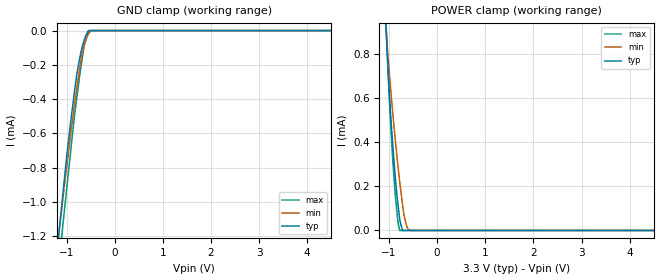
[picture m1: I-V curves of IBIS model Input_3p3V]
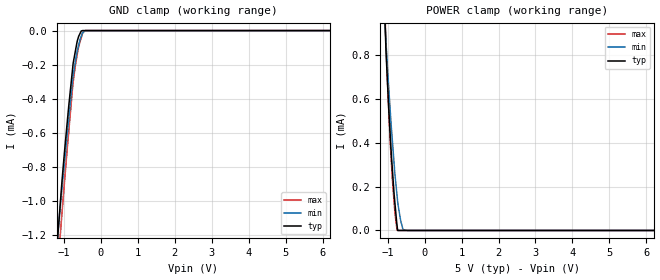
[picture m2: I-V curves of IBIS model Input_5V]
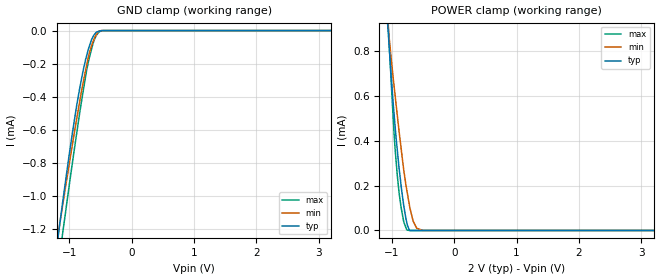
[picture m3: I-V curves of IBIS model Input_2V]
| Texas Instruments Incorporated
| 16-Bit, Quad Channel, Ultra-Low Glitch, Voltage Output DAC with 2.5V,
| 2ppm/C Internal Reference
| Marketing part#   Voltage Range   Package-type   #pins
| DAC8564IAPW   1.8 to 5.5V   TSSOP   16
| DAC8564IAPWG4   1.8 to 5.5V   TSSOP   16
| DAC8564IAPWR   1.8 to 5.5V   TSSOP   16
| DAC8564IAPWRG4   1.8 to 5.5V   TSSOP   16
| DAC8564IBPW   1.8 to 5.5V   TSSOP   16
| DAC8564IBPWG4   1.8 to 5.5V   TSSOP   16
| DAC8564IBPWR   1.8 to 5.5V   TSSOP   16
| DAC8564IBPWRG4   1.8 to 5.5V   TSSOP   16
| DAC8564ICPW   1.8 to 5.5V   TSSOP   16
| DAC8564ICPWG4   1.8 to 5.5V   TSSOP   16
| DAC8564ICPWR   1.8 to 5.5V   TSSOP   16
| DAC8564ICPWRG4   1.8 to 5.5V   TSSOP   16
| DAC8564IDPW   1.8 to 5.5V   TSSOP   16
| DAC8564IDPWG4   1.8 to 5.5V   TSSOP   16
| DAC8564IDPWR   1.8 to 5.5V   TSSOP   16
| DAC8564IDPWRG4   1.8 to 5.5V   TSSOP   16
[IBIS Ver]   3.2
[File name]   dac8564.ibs
|SIMDE Ver   V2.0 - 201002 - RHL4 - Build 372
[Date]   29 July 2010
[File Rev]   1.2
[Source]
| Texas Instruments Incorporated.
| Analog eLab Design Center, HPA
| 12500 TI Blvd
| Dallas, TX -75243
| e-Mail: elab_scm_ibis@list.ti.com
| Model generated from simulations in TISPICE
[Notes]Revision_History:
|   Rev 1.0: 06/08/2010
|   - Initial version of the model
|   - Model names with a trailing _2p25V stands for the Model
|   with typical voltage 2.25V -[1.8V,2.25V,2.7V].Model names
|   with a trailing _4p1V stands for the Model with typical
|   voltage 4.1V-[2.7V,4.1V,5.5V]
|   Rev 1.1: 07/08/2010
|   - Model generated from simulations in TISPICE
|   - Model matched to SPICE simulation
|   - Updated the ibis file with data sheet title and package
|   details
|   - While calculating R_pkg, L_pkg and C_pkg ignored values
|   corresponding to power and ground pins
|   - Added package details beside [Package]
|   - Re-genearted the Models with std typical values of 3.3V
|   and 5V . The 2 Models are
|   1) Input_3p3V - corresponds to 3V  , 3.3V,3.6V
|   2) Input_5V   - corresponds to 4.5V, 5V  ,5.5V
|   - C_comp although listed in numerical order of value are
|   obtained from varying PVT conditions. For PVT conditions
|   for each specific value refer the buffer description under
|   respective [Model]. IBIS model user is responsible for using
|   appropriate C_comp to simulate for Signal Integrity
|   Rev 1.2: 07/08/2010
|   - Corrected Vinl and Vinh for all models
|   - Removed all points beyond rail voltages
|   - Used 1.0E-20F for C_comp of TERM
|   - Corrected the typical value calculation for package RLC
[Disclaimer]
| This model is designed as an aid for customers of Texas Instruments.
| TI and its licensors and suppliers make no warranties, either expressed
| or implied, with respect to this  model, including the warranties of
| merchantability or fitness for a particular purpose. The model is
| provided solely on an "as is" basis. The entire risk as to its quality
| and performance is with the customer.
[Copyright]
| (C) Copyright 2010 Texas Instruments Incorporated. All rights reserved.
|   DAC8564
[Component]   DAC8564
[Manufacturer]  TI
[Package] | 16 TSSOP - PW package
|   typ   min   max
R_pkg   0.05811   0.02779   0.08182
L_pkg   2.21350E-09   1.70135E-09   2.86250E-09
C_pkg   0.47245E-12   0.44143E-12   0.51313E-12
|-------------------------PINS------------------------------------------------
[Pin]  signal_name   model_name   R_pin   L_pin   C_pin
1   VOUT_A   NC   0.04433   2.55695E-09   0.51313E-12
2   VOUT_B   NC   0.04120   1.94352E-09   0.46611E-12
3   VREF_H/VREF_OUT term   0.02779   1.70135E-09   0.50494E-12
4   AVDD   POWER   0.02688   1.68698E-09   0.49746E-12
5   VREF_L   term   0.03604   1.75816E-09   0.47239E-12
6   GND   GND   0.02752   1.74852E-09   0.49261E-12
7   VOUT_C   NC   0.04259   1.98332E-09   0.46901E-12
8   VOUT_D   NC   0.04432   2.56006E-09   0.51267E-12
9   _SYNC   Input   0.07777   2.80109E-09   0.49072E-12
10   SCLK   Input   0.07962   2.26331E-09   0.44148E-12
11   DIN   Input   0.06860   2.06333E-09   0.44715E-12
12   IOVDD   POWER   0.03580   1.75989E-09   0.46496E-12
13   A0   Input   0.06309   1.96557E-09   0.44143E-12
14   A1   Input   0.06860   2.05920E-09   0.44679E-12
15   _ENABLE   Input   0.07962   2.25708E-09   0.44154E-12
16   LDAC   Input   0.08182   2.86250E-09   0.49444E-12
|   Model Selectors
[Model selector] Input
 Input_3p3V   3.3V nominal input
 Input_5V   5V   nominal input
 Input_2V   2V nominal input
|NOTES   Model Selector is used to select between the Input Models which
|   have 3 Voltage ranges namely
|   1) Input_2V   -  1.8,2,2.2V
|   2) Input_3p3V -  3,3.3,3.6V
|   3) Input_5V   -  4.5,5,5.5V
[Model selector] term
 term_3p3V  3.3V nominal termination
 term_5V   5V   nominal termination
 term_2V   2V   nominal termination
|   Termination - term_3p3V
[Model] term_3p3V
Model_type Terminator
C_comp  1.0E-20F 1.0E-20F 1.0E-20F
| variable   typ   min   max
[Voltage Range]   3.30000v  3.00000V  3.60000V
[POWER Clamp Reference]  3.30000v  3.00000V  3.60000V
[GND Clamp Reference]   0.00000V  0.00000V  0.00000V
[Temperature Range]   25   105   -40
|   Termination - term_5V
[Model] term_5V
Model_type Terminator
C_comp  1.0E-20F 1.0E-20F 1.0E-20F
| variable   typ   min   max
[Voltage Range]   5.00000V  4.50000V  5.50000V
[POWER Clamp Reference]  5.00000V  4.50000V  5.50000V
[GND Clamp Reference]   0.00000V  0.00000V  0.00000V
[Temperature Range]   25   105   -40
|   Termination - term_2V
[Model] term_2V
Model_type Terminator
C_comp  1.0E-20F 1.0E-20F 1.0E-20F
| variable   typ   min   max
[Voltage Range]   2.00000V  1.80000V  2.20000V
[POWER Clamp Reference]  2.00000V  1.80000V  2.20000V
[GND Clamp Reference]   0.00000V  0.00000V  0.00000V
[Temperature Range]   25   105   -40
| Models and submodels in the file (6): Input_3p3V (Input), Input_5V (Input), Input_2V (Input), term_3p3V (Terminator), term_5V (Terminator), term_2V (Terminator)
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|NOTES   Three separate Terminators are modelled for the 3 range of
|   voltages
|   1) term_3p3V -  3,3.3,3.6V
|   2) term_5V   -  4.5,5,5.5V
|   3) term_2p5V -  1.8,2,2.2V
|   Model   - Input_3p3V
[Model]   Input_3p3V
Model_type   Input
Vinl = 0.99
Vinh = 2.31
|   typ   min   max
|   (nom PVT)   (Fast PVT)   (slow PVT)
C_comp   4.648e-13   4.575e-13   5.349e-13
| Where   nom  PVT is  Nominal Process, 3.3V, 25C
|   Fast PVT is Strong Process, 3.6V, -40C
|   Slow PVT is Weak Process, 3.0V, 105C
[model spec]
Vinl   0.99   0.9   1.08
Vinh   2.31   2.1   2.52
[Voltage Range]   3.3   3   3.6
|Ambient Temperature   25   105   -40
|Junction Temperature
[Temperature Range]   25   105   -40
[Power Clamp Reference]   3.3   3   3.6
[GND Clamp Reference]   0   0   0
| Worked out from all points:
|   GND clamp passes 1 mA (typ) near -1.09 V on its own axis
|   POWER clamp passes 1 mA (typ) near -1.08 V on its own axis
[GND Clamp]
|   Voltage   I(typ)   I(min)   I(max)
-3.3V     -7.771mA   -6.599mA   -9.241mA
-1.178V   -1.239mA   -1.228mA   -1.424mA
-1.079V   -961uA     -989.1uA   -1.143mA
-986.7mV  -708.8uA   -773.2uA   -897.2uA
-910.8mV  -524.5uA   -596.9uA   -694.5uA
-834mV    -353.1uA   -431.1uA   -497.2uA
-785.4mV  -253uA     -332.6uA   -390.9uA
-693mV    -117.5uA   -156.6uA   -198.1uA
-636mV    -59.22uA   -87.82uA   -94.01uA
-549.6mV  -492.7nA   -23.01uA   -15.28uA
-471.9mV  0A         0A         0A
6.6V      0A         0A         0A
[POWER Clamp]
|   Voltage   I(typ)   I(min)   I(max)
-3.3V     13.63mA    11.23mA    16.39mA
-1.076V   970.6uA    953.2uA    1.029mA
-1.036V   801.6uA    830uA      786.9uA
-983.4mV  583.8uA    687.3uA    551.2uA
-916.8mV  371.6uA    519.3uA    300uA
-866.4mV  233.2uA    401.4uA    151.6uA
-816mV    122.3uA    293.9uA    42.15uA
-778.8mV  53.33uA    221.7uA    0A
-719.4mV  0A         118.1uA    0A
-672mV    0A         53.15uA    0A
-546mV    0A         0A         0A
6.6V      0A         0A         0A
|   Model   - Input_5V
[Model]   Input_5V
Model_type   Input
Vinl = 1.5
Vinh = 3.5
|   typ   min   max
|   (nom PVT)   (Fast PVT)   (slow PVT)
C_comp   4.340e-13   3.990e-13   5.345e-13
| Where   nom  PVT is  Nominal Process, 5V, 25C
|   Fast PVT is Strong Process, 5.5V, -40C
|   Slow PVT is Weak Process, 4.5V, 105C
[model spec]
Vinl   1.5   1.35   1.65
Vinh   3.5   3.15   3.85
[Voltage Range]   5   4.5   5.5
|Ambient Temperature   25   105   -40
|Junction Temperature
[Temperature Range]   25   105   -40
[Power Clamp Reference]   5   4.5   5.5
[GND Clamp Reference]   0   0   0
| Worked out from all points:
|   GND clamp passes 1 mA (typ) near -1.09 V on its own axis
|   POWER clamp passes 1 mA (typ) near -1.08 V on its own axis
[GND Clamp]
|   Voltage   I(typ)   I(min)   I(max)
-5V       -13.07mA   -10.95mA   -15.71mA
-1.155V   -1.177mA   -1.174mA   -1.362mA
-1.079V   -959.1uA   -987.9uA   -1.144mA
-990mV    -726.1uA   -787.4uA   -903.6uA
-870mV    -444.5uA   -519.3uA   -594.1uA
-750mV    -191.7uA   -263.6uA   -301.6uA
-640mV    -62.84uA   -120.2uA   -140.6uA
-600mV    -33uA      -83.78uA   -92.78uA
-530mV    -2.078uA   -32.4uA    -41.23uA
-490mV    0A         -10.72uA   -13.32uA
-423.5mV  0A         0A         0A
10V       0A         0A         0A
[POWER Clamp]
|   Voltage   I(typ)   I(min)   I(max)
-5V       23.6mA     19.51mA    28.37mA
-1.094V   1.06mA     1.017mA    1.141mA
-1.056V   876.4uA    897.1uA    904.7uA
-990.5mV  625.8uA    702.1uA    620uA
-930mV    430uA      543.8uA    402.5uA
-869.5mV  270.8uA    401.9uA    226.7uA
-798mV    114.6uA    247.1uA    72.56uA
-745mV    20.34uA    157.4uA    1.195uA
-729.5mV  581.7nA    131.2uA    0A
-594.5mV  0A         10.2uA     0A
-451.5mV  0A         0A         0A
10V       0A         0A         0A
|   Model   - Input_2V
[Model]   Input_2V
Model_type   Input
Vinl = 0.2
Vinh = 1.9
|   typ   min   max
|   (nom PVT)   (Fast PVT)   (slow PVT)
C_comp   4.997e-13   4.480e-13   5.391e-13
| Where   nom  PVT is  Nominal Process, 2V, 25C
|   Fast PVT is Strong Process, 2.2V, -40C
|   Slow PVT is Weak Process, 1.8V, 105C
[model spec]
Vinl   0.2   0.18   0.22
Vinh   1.9   1.71   2.09
[Voltage Range]   2   1.8   2.2
|Ambient Temperature   25   105   -40
|Junction Temperature
[Temperature Range]   25   105   -40
[Power Clamp Reference]   2   1.8   2.2
[GND Clamp Reference]   0   0   0
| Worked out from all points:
|   GND clamp passes 1 mA (typ) near -1.09 V on its own axis
|   POWER clamp passes 1 mA (typ) near -1.09 V on its own axis
[GND Clamp]
|   Voltage   I(typ)   I(min)   I(max)
-2V       -3.727mA   -3.282mA   -4.306mA
-1.168V   -1.212mA   -1.204mA   -1.397mA
-1.108V   -1.039mA   -1.059mA   -1.228mA
-944mV    -601.3uA   -672.3uA   -780.8uA
-878mV    -443uA     -523.6uA   -608.9uA
-782mV    -247.4uA   -320.5uA   -374.3uA
-721.8mV  -150.5uA   -208.1uA   -237.8uA
-684.4mV  -99.5uA    -143.7uA   -171uA
-620.6mV  -36.88uA   -66.41uA   -78.82uA
-558mV    -7.517uA   -17.35uA   -24.33uA
-454mV    0A         0A         0A
4V        0A         0A         0A
[POWER Clamp]
|   Voltage   I(typ)   I(min)   I(max)
-2V       6.043mA    4.961mA    7.255mA
-1.066V   914uA      922.6uA    963.1uA
-1.041V   809.3uA    851uA      822.9uA
-963.8mV  516.2uA    641.4uA    426.9uA
-913.2mV  358.9uA    513.5uA    246.9uA
-853.8mV  204.4uA    371uA      105.7uA
-807.6mV  108uA      265.3uA    37.1uA
-761.4mV  36.33uA    181.2uA    2.937uA
-718mV    0A         112uA      0A
-657.2mV  0A         40.84uA    0A
-502.4mV  0A         0A         0A
4V        0A         0A         0A
